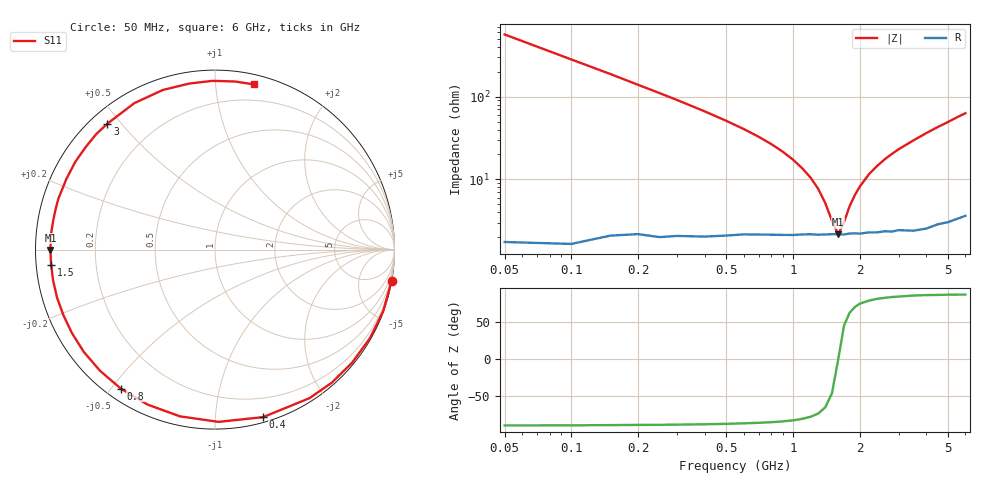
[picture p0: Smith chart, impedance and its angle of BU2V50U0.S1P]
! Infineon Technologies  Discrete & RF Semiconductors
! BB 833
! Si Tuning Diode in SOD323
! VR = 2.5 V
! S-Parameters:  June  1999
# GHz  S  MA  R  50
!  f  S11
! GHz  MAG  ANG
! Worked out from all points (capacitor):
!   34 points, 50 MHz to 6 GHz, reference 50 ohm
!   read as one part to ground: C = 5.62 pF near 50 MHz
!   lowest |Z| = 2.17 ohm at 1.6 GHz (marker M1)
!   series resonance near 1.602 GHz, so ESL is about 1.8 nH
!   S11 on the Smith chart (normalised r, x): 50 MHz: 0, -11; 400 MHz: 0.04, -1.33; 800 MHz: 0.04, -0.53; 1.5 GHz: 0.04, -0.05; 3 GHz: 0.05, +0.46; 6 GHz: 0.07, +1.26
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0.05  0.9995 -10.1
0.1  0.998 -20.1
0.15  0.9945 -29.8
0.2  0.9901 -39.5
0.25  0.9865 -48.7
0.3  0.9811 -57.5
0.4  0.9711 -74.0
0.5  0.9599 -88.8
0.6  0.9493 -101.9
0.7  0.9417 -113.6
0.8  0.9355 -124.1
0.9  0.9307 -133.5
1  0.927 -142.0
1.1  0.9229 -149.8
1.3  0.9198 -163.2
1.5  0.9171 -174.8
1.6  0.917 -179.9
1.8  0.916 170.5
2  0.9176 162.2
2.4  0.9192 147.9
2.8  0.923 135.9
3  0.923 130.5
3.5  0.9316 118.8
4  0.9356 108.1
4.5  0.9362 98.8
5  0.9404 90.8
5.5  0.9431 83.2
6  0.9457 76.8
